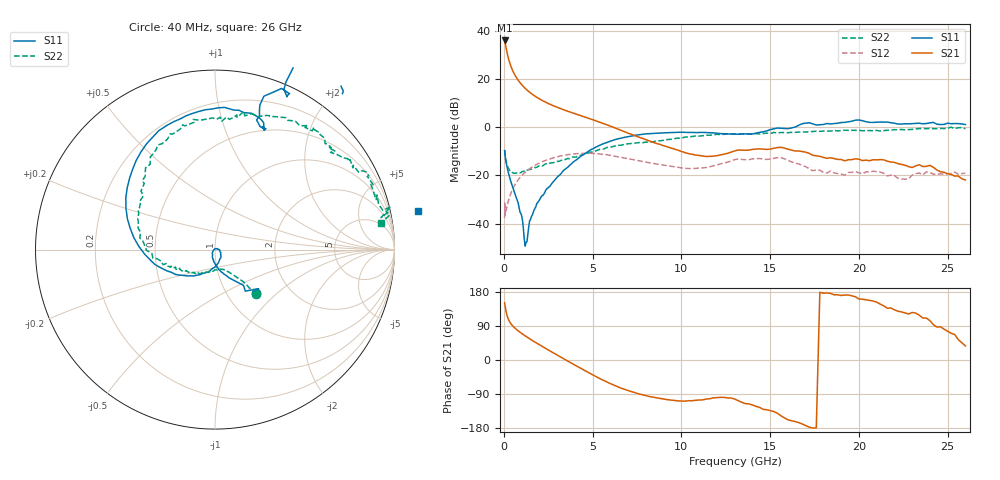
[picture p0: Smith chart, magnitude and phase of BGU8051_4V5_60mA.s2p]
! BGU8051_4V5_60mA
! Date/time Tue Jun 16 11:13:39 2015
! VAR V_out= 4.5000
! VAR I_out= 59.9150
! VAR V_in= 6.3960
! VAR I_in= 0.8257
# MHz S MA R 50
!  Freq-MHz  S11-mag  S11-arg  S21-mag  S21-arg  S12-mag  S12-arg  S22-mag  S22-arg
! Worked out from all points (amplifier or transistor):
!   197 points, 40 MHz to 26 GHz, reference 50 ohm
!   highest |S21| = 36.2 dB at 40 MHz (marker M1)
!   |S21| within 3 dB of that: start of sweep to 119.9 MHz
!   unconditionally stable (mu >= 1): 314.8 MHz to 13.29 GHz; 13.47 GHz to 14.01 GHz
!   at 800 MHz: K = 1.02, MAG = 19.9 dB, |S12| = -21.9 dB
!   at 6.4 GHz: K = 1.30, MAG = 2.5 dB, |S12| = -12.1 dB
!   at 26 GHz: K = -1.07, MSG = -1.4 dB, |S12| = -19.0 dB
!   lowest NFmin = 0.41 dB at 400 MHz
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40  0.3308 -47.0  64.36 151.0  0.01294 32.8  0.3356 -46.8
60  0.2865 -53.9  59.33 145.0  0.01674 14.2  0.2878 -48.2
80  0.242 -52.8  54.04 139.0  0.01599 38.6  0.2411 -48.6
120  0.1941 -59.6  45.55 128.3  0.01892 45.6  0.1999 -51.5
160  0.1614 -65.7  38.48 120.1  0.02139 51.4  0.1749 -54.0
200  0.1373 -71.3  32.96 113.8  0.0247 56.3  0.1571 -57.1
260  0.1117 -79.9  26.93 106.6  0.03011 59.4  0.1393 -60.5
320  0.09088 -84.5  22.59 101.1  0.03559 61.0  0.1282 -63.6
400  0.0725 -92.3  18.5 95.4  0.04359 62.7  0.1207 -67.3
500  0.05706 -98.6  15.06 89.8  0.05279 63.2  0.1151 -73.2
700  0.03475 -112.8  10.96 80.9  0.07137 61.4  0.1119 -81.3
900  0.01771 -134.5  8.601 73.5  0.08987 58.4  0.1127 -90.6
1200  0.003384 159.0  6.492 63.7  0.1167 52.9  0.1208 -101.6
1550  0.01396 25.2  5.05 53.1  0.1465 45.9  0.1357 -112.1
2700  0.06819 -70.3  2.913 21.2  0.2283 20.6  0.1839 -138.2
4400  0.2616 -148.3  1.719 -23.8  0.2891 -18.0  0.2658 -158.3
6600  0.5991 144.6  0.8675 -74.2  0.238 -60.4  0.4256 166.8
8800  0.7626 102.2  0.4424 -101.3  0.1696 -78.3  0.5267 141.1
13200  0.7177 67.6  0.3389 -107.3  0.2199 -91.7  0.7318 92.2
17400  1.188 49.7  0.2632 -179.4  0.125 -156.3  0.8209 64.1
21800  1.25 24.0  0.1905 137.3  0.1018 -171.3  0.8783 35.6
26000  1.148 10.7  0.08054 37.1  0.1117 173.3  0.9379 9.2
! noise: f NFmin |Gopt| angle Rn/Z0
400  0.4144  0.01542  252.2  0.0507
550  0.4211  0.02842  207.7  0.0505
950  0.4516  0.07352  190  0.0501
1250  0.4865  0.1028  188.7  0.0502
1600  0.5402  0.1316  189.8  0.0508
1900  0.5974  0.1525  191.7  0.0521
2250  0.6772  0.1736  194.6  0.0547
2600  0.7709  0.1925  198.2  0.0588
3300  1.001  0.2292  206.5  0.0725
4000  1.286  0.2725  214.9  0.0955
